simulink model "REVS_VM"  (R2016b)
settings: Solver=ode3  StartTime=REVS.sim_start_time_secs  StopTime=Inf  FixedStep=REVS.sim_step_time_secs  MaxStep=REVS.sim_step_time_secs  EnableMultiTasking=on
StopFcn:
  | postproc_datalog;
  | postproc_audit;
  | postproc_result;
model workspace (MATLAB code in the model file):
  other statements: REVS_setup_variants
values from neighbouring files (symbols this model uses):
  accessory = class_accessory_data    [class_test_data.m]
  battery = class_battery_data    [class_accessory_data.m]    (also in class_REVS_electric.m = class_REVS_battery)
  brake = struct(	'max_torque_Nm',[], 						'proportion_norm',1.0, 						'inertia_kgm2',0.0)    [class_REVS_drive_axle.m]
  engine = class_engine_data    [class_test_data.m]
  final_drive = struct(	'gear_ratio',[], 								'efficiency_norm',[], 								'inertia_kgm2',[] )    [class_REVS_drive_axle.m]
  gear = class_REVS_gearbox    [class_REVS_AT_transmission.m]
  tire = struct(	'radius_m',[], 						'rolling_resistance_coefficient',0, 						'vehicle_weight_norm',1.0,  						'wheel_slip_torque_Nm',[],  						'inertia_kgm2',0.0)    [class_REVS_drive_axle.m]
  torque_converter = class_REVS_torque_converter    [class_REVS_AT_transmission.m]
  transmission = class_transmission_data    [class_test_data.m]
  vehicle = class_vehicle_data    [class_test_data.m]
undefined symbols (not defined in the file or in its folder): alternator, ambient, controls, convert, DelayTimeSecs, drive_cycle, driver, electric, gear_strategy, InitialCondition, InitialValue, LoadSource, LookupStructure, MultiplyPosInputs, Normalize, NumPhases, REVS, SpeedSource, starter, tableshift, UpperSaturationLimit, Value, VerboseLevel, VerboseSignal
libraries: simulink x153
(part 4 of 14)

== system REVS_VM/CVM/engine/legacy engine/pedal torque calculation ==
  eng_on : Inport
  eng_spd_radps : Inport  Port=2
  eng_des_acl_norm : Inport  Port=3
  eng_des_load_limit_Nm : Inport  Port=4
  Closed Throttle Torque : Lookup_n-D  NumberOfTableDimensions=1  BreakpointsForDimension1=engine.closed_throttle_speed_radps  BeginIndexSearchUsingPreviousIndexResult=on  Table=engine.closed_throttle_torque_Nm  ExtrapMethod=Clip  UseLastTableValue=on  RndMeth=Simplest
  Full Throttle Torque : Lookup_n-D  NumberOfTableDimensions=1  BreakpointsForDimension1=engine.full_throttle_speed_radps  BeginIndexSearchUsingPreviousIndexResult=on  Table=engine.full_throttle_torque_Nm  ExtrapMethod=Clip  UseLastTableValue=on  RndMeth=Simplest
  MinMax5 : MinMax  Inputs=2  ZeroCross=off
  Pedal Map Torque : Lookup_n-D  BreakpointsForDimension1=engine.pedal_map_pedal_norm  BreakpointsForDimension2=engine.pedal_map_speed_radps  BeginIndexSearchUsingPreviousIndexResult=on  Table=engine.pedal_map_Nm  RndMeth=Simplest
  Product1 : Product
  Product2 : Product
  Product4 : Product  Inputs=3
  Sum : Sum
  to datalog1 : Subsystem
  to datalog2 : Subsystem
  to datalog3 : Subsystem
  to datalog4 : Subsystem
  to datalog5 : Subsystem
  des_pwr_W : Outport
  current_max_pwr_W : Outport  Port=2
  des_trq_Nm : Outport  Port=3
  current_max_trq_Nm : Outport  Port=4
  current_min_trq_Nm : Outport  Port=5
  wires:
  Pedal Map Torque/1 -> Product1/2
  eng_des_load_limit_Nm/1 -> MinMax5/2
  Full Throttle Torque/1 -> current_max_trq_Nm/1, to datalog4/1(Var), Product4/3
  Product4/1 -> current_max_pwr_W/1, to datalog3/1(Var)
  eng_spd_radps/1 -> Product2/1, Closed Throttle Torque/1, Full Throttle Torque/1, Product4/2, Pedal Map Torque/2
  Product2/1 -> to datalog2/1(Var), des_pwr_W/1
  MinMax5/1 -> to datalog1/1(Var), des_trq_Nm/1, Product2/2
  eng_on/1 -> Product4/1, Product1/1
  Closed Throttle Torque/1 -> Sum/1, current_min_trq_Nm/1, to datalog5/1(Var)
  Product1/1 -> Sum/2
  Sum/1 -> MinMax5/1
  eng_des_acl_norm/1 -> Pedal Map Torque/1

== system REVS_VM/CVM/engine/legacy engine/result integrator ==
  in : Inport
  Data Type Conversion : DataTypeConversion  OutDataTypeStr=double
  Integrator1 : Integrator  UpperSaturationLimit=Inf  LowerSaturationLimit=0  ZeroCross=off
  Integrator2 : Integrator  UpperSaturationLimit=Inf  LowerSaturationLimit=0  ZeroCross=off
  Phase To Workspace : ToWorkspace  VariableName=result__phase_fuel_consumed_g  SampleTime=-1
  Product1 : Product  Multiplication=Matrix(*)
  Reshape : Reshape
  Total To Workspace : ToWorkspace  VariableName=result__total_fuel_consumed_g  SampleTime=-1
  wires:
  Reshape/1 -> Integrator1/1, Product1/1
  Data Type Conversion/1 -> Reshape/1
  Integrator2/1 -> Phase To Workspace/1
  [REVS_phase_flag] -> Product1/2
  Product1/1 -> Integrator2/1
  Integrator1/1 -> Total To Workspace/1
  in/1 -> Data Type Conversion/1

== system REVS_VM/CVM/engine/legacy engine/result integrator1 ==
  in : Inport
  Data Type Conversion : DataTypeConversion  OutDataTypeStr=double
  Integrator1 : Integrator  UpperSaturationLimit=Inf  LowerSaturationLimit=0  ZeroCross=off
  Integrator2 : Integrator  UpperSaturationLimit=Inf  LowerSaturationLimit=0  ZeroCross=off
  Phase To Workspace : ToWorkspace  VariableName=result__phase_engine_revolutions  SampleTime=-1
  Product1 : Product  Multiplication=Matrix(*)
  Reshape : Reshape
  Total To Workspace : ToWorkspace  VariableName=result__total_engine_revolutions  SampleTime=-1
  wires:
  Reshape/1 -> Integrator1/1, Product1/1
  Data Type Conversion/1 -> Reshape/1
  Integrator2/1 -> Phase To Workspace/1
  [REVS_phase_flag] -> Product1/2
  Product1/1 -> Integrator2/1
  Integrator1/1 -> Total To Workspace/1
  in/1 -> Data Type Conversion/1

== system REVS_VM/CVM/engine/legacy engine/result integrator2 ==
  in : Inport
  Data Type Conversion : DataTypeConversion  OutDataTypeStr=double
  Integrator1 : Integrator  UpperSaturationLimit=Inf  LowerSaturationLimit=0  ZeroCross=off
  Integrator2 : Integrator  UpperSaturationLimit=Inf  LowerSaturationLimit=0  ZeroCross=off
  Phase To Workspace : ToWorkspace  VariableName=result__phase_engine_running_time_secs  SampleTime=-1
  Product1 : Product  Multiplication=Matrix(*)
  Reshape : Reshape
  Total To Workspace : ToWorkspace  VariableName=result__total_engine_running_time_secs  SampleTime=-1
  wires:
  Reshape/1 -> Integrator1/1, Product1/1
  Data Type Conversion/1 -> Reshape/1
  Integrator2/1 -> Phase To Workspace/1
  [REVS_phase_flag] -> Product1/2
  Product1/1 -> Integrator2/1
  Integrator1/1 -> Total To Workspace/1
  in/1 -> Data Type Conversion/1

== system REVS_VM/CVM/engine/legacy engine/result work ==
  torque_Nm : Inport
  speed_radps : Inport  Port=2
  upstream_iner_kgm2 : Inport  Port=3
  Derivative : Derivative  CoefficientInTFapproximation=1e6
  Gain : Gain  Gain=1/1000
  Integrator1 : Integrator  UpperSaturationLimit=Inf  LowerSaturationLimit=0  ZeroCross=off
  Integrator2 : Integrator  UpperSaturationLimit=Inf  LowerSaturationLimit=0  ZeroCross=off
  Phase To Workspace : ToWorkspace  VariableName=result__phase_crankshaft_output_pos_work_kJ  SampleTime=-1
  Pos : Fcn  Expr=u(1)*(u(1) >= 0)
  Product : Product
  Product1 : Product
  Product2 : Product
  Subtract : Sum  Inputs=+-
  Total To Workspace : ToWorkspace  VariableName=result__total_crankshaft_output_pos_work_kJ  SampleTime=-1
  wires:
  Product2/1 -> Pos/1
  Pos/1 -> Gain/1
  Gain/1 -> Integrator1/1, Product/2
  Product1/1 -> Subtract/2
  Derivative/1 -> Product1/1
  speed_radps/1 -> Derivative/1, Product2/2
  upstream_iner_kgm2/1 -> Product1/2
  Subtract/1 -> Product2/1
  Integrator2/1 -> Phase To Workspace/1
  [REVS_phase_flag] -> Product/1
  Product/1 -> Integrator2/1
  Integrator1/1 -> Total To Workspace/1
  torque_Nm/1 -> Subtract/1

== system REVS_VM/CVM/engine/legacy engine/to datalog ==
  Var : Inport
  Constant : Constant  Value=VerboseSignal
  Constant1 : Constant  Value=VerboseLevel
  Relational Operator : RelationalOperator  OutDataTypeStr=boolean  ZeroCross=off
  Subsystem : Subsystem
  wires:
  Constant1/1 -> Relational Operator/2
  Constant/1 -> Relational Operator/1
  Relational Operator/1 -> Subsystem/Enable
  Var/1 -> Subsystem/1(In1)

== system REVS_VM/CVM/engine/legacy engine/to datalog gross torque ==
  Var : Inport
  Constant : Constant  Value=VerboseSignal
  Constant1 : Constant  Value=VerboseLevel
  Relational Operator : RelationalOperator  OutDataTypeStr=boolean  ZeroCross=off
  Subsystem : Subsystem
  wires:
  Constant1/1 -> Relational Operator/2
  Constant/1 -> Relational Operator/1
  Relational Operator/1 -> Subsystem/Enable
  Var/1 -> Subsystem/1(In1)

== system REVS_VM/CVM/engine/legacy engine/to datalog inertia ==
  Var : Inport
  Constant : Constant  Value=VerboseSignal
  Constant1 : Constant  Value=VerboseLevel
  Relational Operator : RelationalOperator  OutDataTypeStr=boolean  ZeroCross=off
  Subsystem : Subsystem
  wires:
  Constant1/1 -> Relational Operator/2
  Constant/1 -> Relational Operator/1
  Relational Operator/1 -> Subsystem/Enable
  Var/1 -> Subsystem/1(In1)

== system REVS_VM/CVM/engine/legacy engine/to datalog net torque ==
  Var : Inport
  Constant : Constant  Value=VerboseSignal
  Constant1 : Constant  Value=VerboseLevel
  Relational Operator : RelationalOperator  OutDataTypeStr=boolean  ZeroCross=off
  Subsystem : Subsystem
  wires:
  Constant1/1 -> Relational Operator/2
  Constant/1 -> Relational Operator/1
  Relational Operator/1 -> Subsystem/Enable
  Var/1 -> Subsystem/1(In1)

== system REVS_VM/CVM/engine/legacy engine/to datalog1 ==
  Var : Inport
  Constant : Constant  Value=VerboseSignal
  Constant1 : Constant  Value=VerboseLevel
  Relational Operator : RelationalOperator  OutDataTypeStr=boolean  ZeroCross=off
  Subsystem : Subsystem
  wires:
  Constant1/1 -> Relational Operator/2
  Constant/1 -> Relational Operator/1
  Relational Operator/1 -> Subsystem/Enable
  Var/1 -> Subsystem/1(In1)

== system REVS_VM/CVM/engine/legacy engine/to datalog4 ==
  Var : Inport
  Constant : Constant  Value=VerboseSignal
  Constant1 : Constant  Value=VerboseLevel
  Relational Operator : RelationalOperator  OutDataTypeStr=boolean  ZeroCross=off
  Subsystem : Subsystem
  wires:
  Constant1/1 -> Relational Operator/2
  Constant/1 -> Relational Operator/1
  Relational Operator/1 -> Subsystem/Enable
  Var/1 -> Subsystem/1(In1)

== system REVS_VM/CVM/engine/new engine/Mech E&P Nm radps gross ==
  " trq_Nm" : Inport
  spd_radps : Inport  Port=2
  iner_kgm2 : Inport  Port=3
  Compare To Constant : simulink/Logic and Bit Operations/Compare To Constant  relop=>=  const=1  OutDataTypeStr=boolean
  Constant : Constant  Value=VerboseSignal
  Subsystem : Subsystem
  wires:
  Constant/1 -> Compare To Constant/1
  Compare To Constant/1 -> Subsystem/Enable
  iner_kgm2/1 -> Subsystem/3(iner_kgm2)
  spd_radps/1 -> Subsystem/2(spd_radps)
  " trq_Nm"/1 -> Subsystem/1(" trq_Nm")

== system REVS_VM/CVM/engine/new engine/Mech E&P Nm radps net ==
  " trq_Nm" : Inport
  spd_radps : Inport  Port=2
  iner_kgm2 : Inport  Port=3
  Compare To Constant : simulink/Logic and Bit Operations/Compare To Constant  relop=>=  const=1  OutDataTypeStr=boolean
  Constant : Constant  Value=VerboseSignal
  Subsystem : Subsystem
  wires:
  Constant/1 -> Compare To Constant/1
  Compare To Constant/1 -> Subsystem/Enable
  iner_kgm2/1 -> Subsystem/3(iner_kgm2)
  spd_radps/1 -> Subsystem/2(spd_radps)
  " trq_Nm"/1 -> Subsystem/1(" trq_Nm")

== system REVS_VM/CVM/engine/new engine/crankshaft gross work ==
  torque_Nm : Inport
  speed_radps : Inport  Port=2
  upstream_iner_kgm2 : Inport  Port=3
  Derivative : Derivative  CoefficientInTFapproximation=1e6
  Gain : Gain  Gain=1/1000
  Integrator1 : Integrator  UpperSaturationLimit=Inf  LowerSaturationLimit=0  ZeroCross=off
  Integrator2 : Integrator  UpperSaturationLimit=Inf  LowerSaturationLimit=0  ZeroCross=off
  Phase To Workspace : ToWorkspace  VariableName=result__phase_crankshaft_gross_pos_work_kJ  SampleTime=-1
  Pos : Fcn  Expr=u(1)*(u(1) >= 0)
  Product : Product
  Product1 : Product
  Product2 : Product
  Subtract : Sum  Inputs=+-
  Total To Workspace : ToWorkspace  VariableName=result__total_crankshaft_gross_pos_work_kJ  SampleTime=-1
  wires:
  Product2/1 -> Pos/1
  Pos/1 -> Gain/1
  Gain/1 -> Integrator1/1, Product/2
  Product1/1 -> Subtract/2
  Derivative/1 -> Product1/1
  speed_radps/1 -> Derivative/1, Product2/2
  upstream_iner_kgm2/1 -> Product1/2
  Subtract/1 -> Product2/1
  Integrator2/1 -> Phase To Workspace/1
  [REVS_phase_flag] -> Product/1
  Product/1 -> Integrator2/1
  Integrator1/1 -> Total To Workspace/1
  torque_Nm/1 -> Subtract/1

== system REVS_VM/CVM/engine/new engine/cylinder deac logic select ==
  note: 1) Only subsystems can be added as variant choices at this level 2) Blocks cannot be connected at this level as connectivity is automatically determined at simulation, based on the active variant
  system_bus : Inport
  constant : Subsystem  VariantControl=get_REVS_engine_deac_strategy_type( engine) == enum_engine_deac_select.constant
  dynamic criteria : Subsystem  VariantControl=get_REVS_engine_deac_strategy_type( engine) == enum_engine_deac_select.dynamic_criteria
  dynamic lookup : Subsystem  VariantControl="get_REVS_engine_deac_strategy_type( engine) ==  enum_engine_deac_select.dynamic_lookup"
  cyl_deac_norm : Outport

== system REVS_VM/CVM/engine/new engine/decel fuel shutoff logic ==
  system_bus : Inport
  eng_rqst_torque_Nm : Inport  Port=2
  eng_load_norm : Inport  Port=3
  Constant : Constant  Value=engine.max_torque_Nm
  Divide : Product  Inputs=*/
  Logical Operator : Logic  Inputs=3  AllPortsSameDT=off  OutDataTypeStr=boolean
  Relay : Relay  OnSwitchValue=0.01  OffSwitchValue=0.005  OnOutputValue=0  OffOutputValue=1  ZeroCross=off
  Relay1 : Relay  OnSwitchValue=0.01  OffSwitchValue=0.005  OnOutputValue=0  OffOutputValue=1  ZeroCross=off
  dynamic equation : Subsystem
  to datalog4 : Subsystem
  dfco_active_bool : Outport
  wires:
  Relay1/1 -> Logical Operator/3
  eng_load_norm/1 -> Relay1/1
  Divide/1 -> Relay/1
  Constant/1 -> Divide/2
  eng_rqst_torque_Nm/1 -> Divide/1
  Relay/1 -> Logical Operator/2
  Logical Operator/1 -> dfco_active_bool/1, to datalog4/1(Var)
  system_bus/1 -> dynamic equation/1(bus)
  dynamic equation/1(out) -> Logical Operator/1

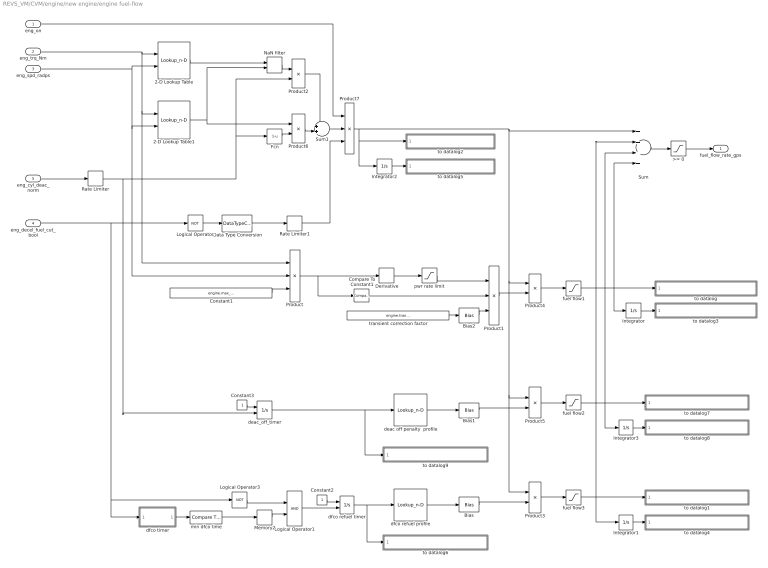
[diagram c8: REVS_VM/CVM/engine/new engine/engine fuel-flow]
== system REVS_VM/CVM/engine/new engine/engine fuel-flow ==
  eng_on : Inport
  eng_trq_Nm : Inport  Port=2
  eng_spd_radps : Inport  Port=3
  eng_decel_fuel_cut_bool : Inport  Port=4
  eng_cyl_deac_norm : Inport  Port=5
  2-D Lookup Table : Lookup_n-D  BreakpointsForDimension1=engine.fuel_map_torque_Nm  BreakpointsForDimension2=engine.fuel_map_speed_radps  IndexSearchMethod=Linear search  BeginIndexSearchUsingPreviousIndexResult=on  Table=engine.deac_fuel_map_gps  ExtrapMethod=Clip  UseLastTableValue=on  RndMeth=Simplest
  2-D Lookup Table1 : Lookup_n-D  BreakpointsForDimension1=engine.fuel_map_torque_Nm  BreakpointsForDimension2=engine.fuel_map_speed_radps  IndexSearchMethod=Linear search  BeginIndexSearchUsingPreviousIndexResult=on  Table=engine.fuel_map_gps  ExtrapMethod=Clip  UseLastTableValue=on  RndMeth=Simplest
  >= 0 : Saturate  UpperLimit=Inf  LowerLimit=0  ZeroCross=off
  Bias : Bias  Bias=-1
  Bias1 : Bias  Bias=-1
  Bias2 : Bias  Bias=-1
  Compare To Constant1 : simulink/Logic and Bit Operations/Compare To Constant  relop=>  const=0  OutDataTypeStr=boolean  ZeroCross=off
  Constant1 : Constant  Value=engine.max_power_W
  Constant2 : Constant
  Constant3 : Constant
  Data Type Conversion : DataTypeConversion  OutDataTypeStr=double
  Derivative : Derivative
  Fcn : Fcn  Expr=1-u
  Integrator{,1..3} (4 alike) : Integrator
  Logical Operator : Logic  Operator=NOT  AllPortsSameDT=off  OutDataTypeStr=boolean
  Logical Operator3 : Logic  Operator=NOT  AllPortsSameDT=off  OutDataTypeStr=boolean
  Logical Operator1 : Logic  AllPortsSameDT=off  OutDataTypeStr=boolean
  Memory2 : Memory
  NaN filter : MinMax  Inputs=2
  Product : Product  Inputs=**/
  Product1 : Product  Inputs=3
  Product{2..6} (5 alike) : Product
  Product7 : Product  Inputs=3
  Rate Limiter : RateLimiter  RisingSlewLimit=1/engine.deac_transition_on_duration_secs  FallingSlewLimit=-1/engine.deac_transition_off_duration_secs  SampleTimeMode=inherited
  Rate Limiter1 : RateLimiter  RisingSlewLimit=5  FallingSlewLimit=-3  SampleTimeMode=inherited
  Sum : Sum  Inputs=++++
  Sum1 : Sum  Inputs=++|
  deac off penalty  profile : Lookup_n-D  NumberOfTableDimensions=1  BreakpointsForDimension1=engine.deac_transition_off_fuel_multiplier_time_secs  IndexSearchMethod=Linear search  BeginIndexSearchUsingPreviousIndexResult=on  Table=engine.deac_transition_off_fuel_multiplier  ExtrapMethod=Clip  RndMeth=Simplest
  deac_off_timer : Integrator  ExternalReset=level
  dfco refuel timer : Integrator  ExternalReset=rising
  dfco refuel profile : Lookup_n-D  NumberOfTableDimensions=1  BreakpointsForDimension1=engine.DFCO_refuel_multiplier_time_secs  IndexSearchMethod=Linear search  BeginIndexSearchUsingPreviousIndexResult=on  Table=engine.DFCO_refuel_multiplier  ExtrapMethod=Clip  RndMeth=Simplest
  dfco timer : Subsystem
  fuel flow1 : Saturate  UpperLimit=inf  LowerLimit=0  ZeroCross=off
  fuel flow2 : Saturate  UpperLimit=engine.deac_transition_off_fuel_multiplier_limit_gps  LowerLimit=0  ZeroCross=off
  fuel flow3 : Saturate  UpperLimit=engine.DFCO_refuel_multiplier_limit_gps  LowerLimit=0  ZeroCross=off
  min dfco time : simulink/Logic and Bit Operations/Compare To Constant  relop=>=  const=engine.DFCO_min_duration_secs  OutDataTypeStr=boolean  ZeroCross=off
  pwr rate limit : Saturate  UpperLimit=0.4  LowerLimit=0  ZeroCross=off
  to datalog : Subsystem
  to datalog1 : Subsystem
  to datalog2 : Subsystem
  to datalog3 : Subsystem
  to datalog4 : Subsystem
  to datalog5 : Subsystem
  to datalog6 : Subsystem
  to datalog7 : Subsystem
  to datalog8 : Subsystem
  to datalog9 : Subsystem
  transient correction factor : Constant  Value=engine.transient_correction_mult
  fuel_flow_rate_gps : Outport
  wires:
  Data Type Conversion/1 -> Rate Limiter1/1
  Rate Limiter1/1 -> Product7/3
  eng_cyl_deac_norm/1 -> Rate Limiter/1
  Bias1/1 -> Product5/2
  deac_off_timer/1 -> deac off penalty  profile/1, to datalog9/1(Var)
  Rate Limiter/1 -> deac_off_timer/2, Fcn/1, Product2/2
  Constant3/1 -> deac_off_timer/1
  deac off penalty  profile/1 -> Bias1/1
  Integrator3/1 -> to datalog8/1(Var)
  Product7/1 -> Integrator2/1, to datalog2/1(Var), Sum/1, Product4/1, Product3/1, Product5/1
  Product5/1 -> fuel flow2/1
  fuel flow2/1 -> to datalog7/1(Var), Sum/3, Integrator3/1
  Sum1/1 -> Product7/2
  Logical Operator3/1 -> Logical Operator1/1
  Logical Operator/1 -> Data Type Conversion/1
  NaN filter/1 -> Product2/1
  Fcn/1 -> Product6/2
  Product2/1 -> Sum1/1
  Product6/1 -> Sum1/2
  2-D Lookup Table1/1 -> NaN filter/2, Product6/1
  Bias/1 -> Product3/2
  dfco refuel profile/1 -> Bias/1
  dfco refuel timer/1 -> dfco refuel profile/1, to datalog6/1(Var)
  Constant2/1 -> dfco refuel timer/1
  Integrator2/1 -> to datalog5/1(Var)
  Derivative/1 -> pwr rate limit/1
  Constant1/1 -> Product/3
  Bias2/1 -> Product1/3
  Product1/1 -> Product4/2
  Integrator1/1 -> to datalog4/1(Var)
  Integrator/1 -> to datalog3/1(Var)
  fuel flow1/1 -> Integrator/1, to datalog/1(Var), Sum/4
  Product4/1 -> fuel flow1/1
  transient correction factor/1 -> Bias2/1
  pwr rate limit/1 -> Product1/1
  Product/1 -> Derivative/1, Compare To Constant1/1
  eng_trq_Nm/1 -> 2-D Lookup Table/1, 2-D Lookup Table1/1, Product/1
  Compare To Constant1/1 -> Product1/2
  eng_spd_radps/1 -> 2-D Lookup Table/2, 2-D Lookup Table1/2, Product/2
  eng_on/1 -> Product7/1
  2-D Lookup Table/1 -> NaN filter/1
  >= 0/1 -> fuel_flow_rate_gps/1
  dfco timer/1(out) -> min dfco time/1
  min dfco time/1 -> Memory2/1
  Memory2/1 -> Logical Operator1/2
  Logical Operator1/1 -> dfco refuel timer/2
  Sum/1 -> >= 0/1
  Product3/1 -> fuel flow3/1
  fuel flow3/1 -> to datalog1/1(Var), Sum/2, Integrator1/1
  eng_decel_fuel_cut_bool/1 -> Logical Operator/1, Logical Operator3/1, dfco timer/1(bool)

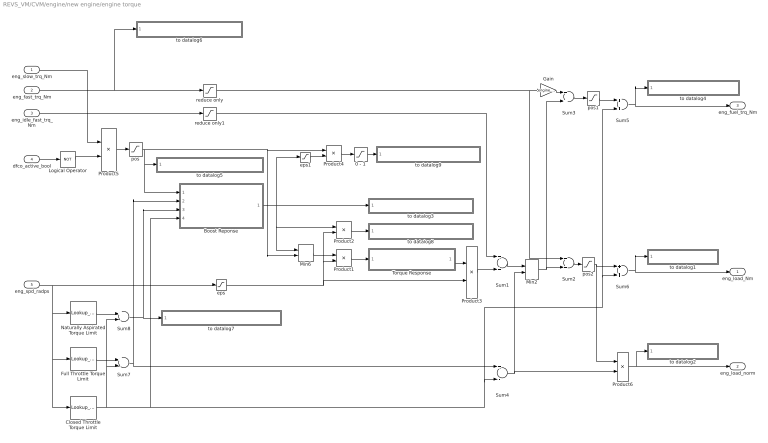
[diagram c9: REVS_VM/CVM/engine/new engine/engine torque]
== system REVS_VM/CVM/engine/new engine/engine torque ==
  eng_slow_trq_Nm : Inport
  eng_fast_trq_Nm : Inport  Port=2
  eng_idle_fast_trq_Nm : Inport  Port=3
  dfco_active_bool : Inport  Port=4
  eng_spd_radps : Inport  Port=5
  0 - 1 : Saturate  UpperLimit=1  LowerLimit=0  ZeroCross=off
  Boost Reponse : Subsystem
  Closed Throttle Torque Limit : Lookup_n-D  NumberOfTableDimensions=1  BreakpointsForDimension1=engine.closed_throttle_speed_radps  BeginIndexSearchUsingPreviousIndexResult=on  Table=engine.closed_throttle_torque_Nm  ExtrapMethod=Clip  UseLastTableValue=on  RndMeth=Simplest
  Full Throttle Torque Limit : Lookup_n-D  NumberOfTableDimensions=1  BreakpointsForDimension1=engine.full_throttle_speed_radps  BeginIndexSearchUsingPreviousIndexResult=on  Table=engine.full_throttle_torque_Nm  ExtrapMethod=Clip  UseLastTableValue=on  RndMeth=Simplest
  Gain : Gain  Gain=engine.fast_torque_fuel_adjust_norm
  Logical Operator : Logic  Operator=NOT  AllPortsSameDT=off  OutDataTypeStr=boolean
  Min2 : MinMax  Inputs=2  ZeroCross=off
  Min6 : MinMax  Inputs=2  ZeroCross=off
  Naturally Aspirated Torque Limit : Lookup_n-D  NumberOfTableDimensions=1  BreakpointsForDimension1=engine.naturally_aspirated_speed_radps  IndexSearchMethod=Linear search  BeginIndexSearchUsingPreviousIndexResult=on  Table=engine.naturally_aspirated_torque_Nm  ExtrapMethod=Clip  UseLastTableValue=on  RndMeth=Simplest
  Product1 : Product
  Product2 : Product
  Product3 : Product  Inputs=*/
  Product4 : Product  Inputs=*/
  Product5 : Product
  Product6 : Product  Inputs=*/
  Sum{1..3,5..6} (5 alike) : Sum
  Sum4 : Sum  Inputs=+-
  Sum7 : Sum  Inputs=+-
  Sum8 : Sum  Inputs=+-
  Torque Response : Subsystem
  eps : Saturate  UpperLimit=inf  LowerLimit=eps
  eps1 : Saturate  UpperLimit=inf  LowerLimit=eps
  pos : Saturate  UpperLimit=inf  LowerLimit=0  ZeroCross=off
  pos1 : Saturate  UpperLimit=inf  LowerLimit=0  ZeroCross=off
  pos2 : Saturate  UpperLimit=inf  LowerLimit=0  ZeroCross=off
  reduce only : Saturate  UpperLimit=0  LowerLimit=-inf  ZeroCross=off
  reduce only1 : Saturate  UpperLimit=0  LowerLimit=-inf  ZeroCross=off
  to datalog1 : Subsystem
  to datalog2 : Subsystem
  to datalog3 : Subsystem
  to datalog4 : Subsystem
  to datalog5 : Subsystem
  to datalog6 : Subsystem
  to datalog7 : Subsystem
  to datalog8 : Subsystem
  to datalog9 : Subsystem
  eng_load_Nm : Outport
  eng_load_norm : Outport  Port=2
  eng_fuel_trq_Nm : Outport  Port=3
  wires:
  pos2/1 -> Product6/1, Sum6/1
  pos1/1 -> Sum5/1
  Sum4/1 -> Product6/2, Min2/2
  Torque Response/1(act_pow_W) -> Product3/1
  Sum3/1 -> pos1/1
  Sum2/1 -> pos2/1
  Logical Operator/1 -> Product5/2
  Product5/1 -> pos/1
  Min2/1 -> Sum2/2, Sum3/2
  dfco_active_bool/1 -> Logical Operator/1
  0 - 1/1 -> to datalog9/1(Var)
  eps1/1 -> Product4/2
  Min6/1 -> Product1/1
  eng_slow_trq_Nm/1 -> Product5/1
  reduce only1/1 -> Sum1/1
  eng_idle_fast_trq_Nm/1 -> reduce only1/1
  Product4/1 -> 0 - 1/1
  eps/1 -> Product1/2, Product2/2, Product3/2
  Product1/1 -> Torque Response/1(target_pow_W)
  Product2/1 -> to datalog8/1(Var)
  Product6/1 -> to datalog2/1(Var), eng_load_norm/1
  Closed Throttle Torque Limit/1 -> Sum8/2, Sum7/2, Sum6/2, Sum5/2, Sum4/2, Boost Reponse/4(min_trq_Nm)
  Sum7/1 -> Sum4/1, Boost Reponse/2(max_trq_Nm)
  Sum8/1 -> Boost Reponse/3(nat_asp_trq_Nm), to datalog7/1(Var)
  pos/1 -> Min6/2, Product4/1, to datalog5/1(Var), Boost Reponse/1(target_trq_Nm)
  Product3/1 -> Sum1/2
  Gain/1 -> Sum3/1
  Sum5/1 -> to datalog4/1(Var), eng_fuel_trq_Nm/1
  Sum1/1 -> Min2/1
  reduce only/1 -> Sum2/1, Gain/1
  eng_fast_trq_Nm/1 -> reduce only/1, to datalog6/1(Var)
  eng_spd_radps/1 -> eps/1, Closed Throttle Torque Limit/1, Full Throttle Torque Limit/1, Naturally Aspirated Torque Limit/1
  Sum6/1 -> to datalog1/1(Var), eng_load_Nm/1
  Boost Reponse/1(trq_limit_Nm) -> to datalog3/1(Var), eps1/1, Product2/1, Min6/1
  Full Throttle Torque Limit/1 -> Sum7/1
  Naturally Aspirated Torque Limit/1 -> Sum8/1

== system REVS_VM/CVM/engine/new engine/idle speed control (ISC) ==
  system_bus : Inport
  eng_spd_radps : Inport  Port=2
  Add : Sum  Inputs=++-
  Closed Throttle Torque : Lookup_n-D  NumberOfTableDimensions=1  BreakpointsForDimension1=engine.closed_throttle_speed_radps  IndexSearchMethod=Linear search  BeginIndexSearchUsingPreviousIndexResult=on  Table=engine.closed_throttle_torque_Nm  ExtrapMethod=Clip  UseLastTableValue=on  RndMeth=Simplest
  Derivative : Derivative
  ISC state : Subsystem
  Idle Speed Target : Subsystem
  PID control : Subsystem
  Split Control Torque : Subsystem
  Sum1 : Sum  Inputs=+-|
  Sum2 : Sum  Inputs=+-
  Taper : Lookup_n-D  NumberOfTableDimensions=1  BreakpointsForDimension1=[-20,-10,0,5,10,15,20]  IndexSearchMethod=Linear search  BeginIndexSearchUsingPreviousIndexResult=on  Table=[-20,-10,0,5,8,10,10]  UseLastTableValue=on  RndMeth=Simplest
  driver bus1 : BusSelector  OutputSignals=powertrain.control.ctrl_eng_on,powertrain.trans.ctrl.eng_des_spd_radps
  eng iner : Gain  Gain=engine.inertia_kgm2
  eng iner2 : Gain  Gain=engine.inertia_kgm2
  gain : Gain  Gain=0.8
  to datalog4 : Subsystem
  to datalog5 : Subsystem
  to datalog6 : Subsystem
  to datalog7 : Subsystem
  to datalog8 : Subsystem
  ISC_state : Outport
  ISC_target_spd_radps : Outport  Port=2
  ISC_slow_trq_Nm : Outport  Port=3
  "ISC_fast_trq_Nm " : Outport  Port=4
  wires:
  Sum1/1 -> Taper/1
  Closed Throttle Torque/1 -> gain/1
  Derivative/1 -> eng iner2/1
  PID control/1(PID_trq_Nm) -> Add/1
  eng iner/1 -> PID control/2(error)
  Add/1 -> Split Control Torque/2(ISC_trq)
  Split Control Torque/2(ISC_fast_trq) -> to datalog8/1(Var), "ISC_fast_trq_Nm "/1
  Split Control Torque/1(ISC_slow_trq) -> ISC_slow_trq_Nm/1, to datalog7/1(Var)
  driver bus1/1 -> ISC state/1(eng_on)  "<ctrl_eng_on>"
  system_bus/1 -> Idle Speed Target/1(system_bus), driver bus1/1
  driver bus1/2 -> Idle Speed Target/3(eng_des_spd_radps)  "<eng_des_spd_radps>"
  ISC state/1(state) -> Idle Speed Target/4(ISC_state), PID control/1(ISC_state), Split Control Torque/1(ISC_state), to datalog6/1(Var), ISC_state/1
  Sum2/1 -> eng iner/1
  eng_spd_radps/1 -> Sum1/2, Closed Throttle Torque/1, Sum2/2, Idle Speed Target/2(eng_spd_radps), ISC state/2(eng_spd_radps)
  Idle Speed Target/1(target_idle_spd_radps) -> Sum1/1, to datalog5/1(Var), ISC_target_spd_radps/1, Sum2/1
  Taper/1 -> Derivative/1
  gain/1 -> Add/3
  eng iner2/1 -> to datalog4/1(Var), Add/2

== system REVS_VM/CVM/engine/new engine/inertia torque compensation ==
  eng_on : Inport
  comp_iner_enable : Inport  Port=2
  eng_spd_radps : Inport  Port=3
  iner_kgm2 : Inport  Port=4
  load_norm : Inport  Port=5
  <= 0 : Saturate  UpperLimit=0  LowerLimit=-Inf  ZeroCross=off
  Memory : Memory
  Product : Product  Inputs=5
  Transfer Fcn : TransferFcn  Numerator=[1 0]  Denominator=[0.02 1]
  downstream compensation : Gain  Gain=1.5
  load based inertia adj. norm : Lookup_n-D  NumberOfTableDimensions=1  BreakpointsForDimension1=[0, 0.65, 0.90, 1.0]  Table=[1.0, 1.0, 0.0, 0.0]  InternalRulePriority=Speed  RndMeth=Simplest
  to datalog1 : Subsystem
  comp_trq_Nm : Outport
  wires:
  comp_iner_enable/1 -> Product/2
  downstream compensation/1 -> Product/4
  Transfer Fcn/1 -> Product/3
  eng_spd_radps/1 -> Transfer Fcn/1
  iner_kgm2/1 -> downstream compensation/1
  <= 0/1 -> to datalog1/1(Var), comp_trq_Nm/1
  eng_on/1 -> Product/1
  load_norm/1 -> Memory/1
  Memory/1 -> load based inertia adj. norm/1
  load based inertia adj. norm/1 -> Product/5
  Product/1 -> <= 0/1

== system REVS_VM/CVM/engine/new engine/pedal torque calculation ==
  eng_on : Inport
  eng_des_acl_norm : Inport  Port=2
  eng_des_load_limit_Nm : Inport  Port=3
  eng_spd_radps : Inport  Port=4
  Closed Throttle Torque : Lookup_n-D  NumberOfTableDimensions=1  BreakpointsForDimension1=engine.closed_throttle_speed_radps  BeginIndexSearchUsingPreviousIndexResult=on  Table=engine.closed_throttle_torque_Nm  ExtrapMethod=Clip  UseLastTableValue=on  RndMeth=Simplest
  MinMax5 : MinMax  Inputs=2  ZeroCross=off
  Pedal Map Torque : Lookup_n-D  BreakpointsForDimension1=engine.pedal_map_pedal_norm  BreakpointsForDimension2=engine.pedal_map_speed_radps  BeginIndexSearchUsingPreviousIndexResult=on  Table=engine.pedal_map_Nm  RndMeth=Simplest
  Product1 : Product
  Product2 : Product
  Sum : Sum
  to datalog1 : Subsystem
  to datalog2 : Subsystem
  to datalog3 : Subsystem
  des_pwr_W : Outport
  des_trq_Nm : Outport  Port=2
  des_gross_trq_Nm : Outport  Port=3
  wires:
  eng_des_load_limit_Nm/1 -> MinMax5/2
  Product1/1 -> MinMax5/1
  MinMax5/1 -> Sum/2, des_gross_trq_Nm/1, to datalog3/1(Var)
  eng_des_acl_norm/1 -> Pedal Map Torque/1
  Closed Throttle Torque/1 -> Sum/1
  eng_on/1 -> Product1/1
  Sum/1 -> des_trq_Nm/1, to datalog1/1(Var), Product2/2
  Product2/1 -> des_pwr_W/1, to datalog2/1(Var)
  eng_spd_radps/1 -> Pedal Map Torque/2, Closed Throttle Torque/1, Product2/1
  Pedal Map Torque/1 -> Product1/2

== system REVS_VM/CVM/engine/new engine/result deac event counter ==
  in : Inport
  Data Type Conversion : DataTypeConversion  OutDataTypeStr=double
  Phase Memory : Memory
  Phase To Workspace : ToWorkspace  VariableName=result__phase_engine_deac_events  SampleTime=-1
  Product : Product
  Sum : Sum  Inputs=|++
  Sum1 : Sum  Inputs=|++
  Total Memory : Memory
  Total To Workspace : ToWorkspace  VariableName=result__total_engine_deac_events  SampleTime=-1
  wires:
  Data Type Conversion/1 -> Product/2, Sum1/1
  Sum1/1 -> Total Memory/1
  Sum/1 -> Phase Memory/1
  in/1 -> Data Type Conversion/1
  Total Memory/1 -> Sum1/2, Total To Workspace/1
  Product/1 -> Sum/1
  [REVS_phase_flag] -> Product/1
  Phase Memory/1 -> Phase To Workspace/1, Sum/2

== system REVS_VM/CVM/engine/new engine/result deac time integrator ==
  in : Inport
  Data Type Conversion : DataTypeConversion  OutDataTypeStr=double
  Integrator1 : Integrator  UpperSaturationLimit=Inf  LowerSaturationLimit=0  ZeroCross=off
  Integrator2 : Integrator  UpperSaturationLimit=Inf  LowerSaturationLimit=0  ZeroCross=off
  Phase To Workspace : ToWorkspace  VariableName=result__phase_engine_deac_time_secs  SampleTime=-1
  Product1 : Product  Multiplication=Matrix(*)
  Reshape : Reshape
  Total To Workspace : ToWorkspace  VariableName=result__total_engine_deac_time_secs  SampleTime=-1
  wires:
  Reshape/1 -> Integrator1/1, Product1/1
  Data Type Conversion/1 -> Reshape/1
  Integrator2/1 -> Phase To Workspace/1
  [REVS_phase_flag] -> Product1/2
  Product1/1 -> Integrator2/1
  Integrator1/1 -> Total To Workspace/1
  in/1 -> Data Type Conversion/1

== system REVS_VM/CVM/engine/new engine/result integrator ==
  in : Inport
  Data Type Conversion : DataTypeConversion  OutDataTypeStr=double
  Integrator1 : Integrator  UpperSaturationLimit=Inf  LowerSaturationLimit=0  ZeroCross=off
  Integrator2 : Integrator  UpperSaturationLimit=Inf  LowerSaturationLimit=0  ZeroCross=off
  Phase To Workspace : ToWorkspace  VariableName=result__phase_fuel_consumed_g  SampleTime=-1
  Product1 : Product  Multiplication=Matrix(*)
  Reshape : Reshape
  Total To Workspace : ToWorkspace  VariableName=result__total_fuel_consumed_g  SampleTime=-1
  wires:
  Reshape/1 -> Integrator1/1, Product1/1
  Data Type Conversion/1 -> Reshape/1
  Integrator2/1 -> Phase To Workspace/1
  [REVS_phase_flag] -> Product1/2
  Product1/1 -> Integrator2/1
  Integrator1/1 -> Total To Workspace/1
  in/1 -> Data Type Conversion/1

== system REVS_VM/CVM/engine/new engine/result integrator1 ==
  in : Inport
  Data Type Conversion : DataTypeConversion  OutDataTypeStr=double
  Integrator1 : Integrator  UpperSaturationLimit=Inf  LowerSaturationLimit=0  ZeroCross=off
  Integrator2 : Integrator  UpperSaturationLimit=Inf  LowerSaturationLimit=0  ZeroCross=off
  Phase To Workspace : ToWorkspace  VariableName=result__phase_engine_revolutions  SampleTime=-1
  Product1 : Product  Multiplication=Matrix(*)
  Reshape : Reshape
  Total To Workspace : ToWorkspace  VariableName=result__total_engine_revolutions  SampleTime=-1
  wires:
  Reshape/1 -> Integrator1/1, Product1/1
  Data Type Conversion/1 -> Reshape/1
  Integrator2/1 -> Phase To Workspace/1
  [REVS_phase_flag] -> Product1/2
  Product1/1 -> Integrator2/1
  Integrator1/1 -> Total To Workspace/1
  in/1 -> Data Type Conversion/1

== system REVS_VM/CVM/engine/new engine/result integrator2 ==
  in : Inport
  Data Type Conversion : DataTypeConversion  OutDataTypeStr=double
  Integrator1 : Integrator  UpperSaturationLimit=Inf  LowerSaturationLimit=0  ZeroCross=off
  Integrator2 : Integrator  UpperSaturationLimit=Inf  LowerSaturationLimit=0  ZeroCross=off
  Phase To Workspace : ToWorkspace  VariableName=result__phase_engine_running_time_secs  SampleTime=-1
  Product1 : Product  Multiplication=Matrix(*)
  Reshape : Reshape
  Total To Workspace : ToWorkspace  VariableName=result__total_engine_running_time_secs  SampleTime=-1
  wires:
  Reshape/1 -> Integrator1/1, Product1/1
  Data Type Conversion/1 -> Reshape/1
  Integrator2/1 -> Phase To Workspace/1
  [REVS_phase_flag] -> Product1/2
  Product1/1 -> Integrator2/1
  Integrator1/1 -> Total To Workspace/1
  in/1 -> Data Type Conversion/1

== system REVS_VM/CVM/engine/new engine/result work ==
  torque_Nm : Inport
  speed_radps : Inport  Port=2
  upstream_iner_kgm2 : Inport  Port=3
  Derivative : Derivative  CoefficientInTFapproximation=1e6
  Gain : Gain  Gain=1/1000
  Integrator1 : Integrator  UpperSaturationLimit=Inf  LowerSaturationLimit=0  ZeroCross=off
  Integrator2 : Integrator  UpperSaturationLimit=Inf  LowerSaturationLimit=0  ZeroCross=off
  Phase To Workspace : ToWorkspace  VariableName=result__phase_crankshaft_output_pos_work_kJ  SampleTime=-1
  Pos : Fcn  Expr=u(1)*(u(1) >= 0)
  Product : Product
  Product1 : Product
  Product2 : Product
  Subtract : Sum  Inputs=+-
  Total To Workspace : ToWorkspace  VariableName=result__total_crankshaft_output_pos_work_kJ  SampleTime=-1
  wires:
  Product2/1 -> Pos/1
  Pos/1 -> Gain/1
  Gain/1 -> Integrator1/1, Product/2
  Product1/1 -> Subtract/2
  Derivative/1 -> Product1/1
  speed_radps/1 -> Derivative/1, Product2/2
  upstream_iner_kgm2/1 -> Product1/2
  Subtract/1 -> Product2/1
  Integrator2/1 -> Phase To Workspace/1
  [REVS_phase_flag] -> Product/1
  Product/1 -> Integrator2/1
  Integrator1/1 -> Total To Workspace/1
  torque_Nm/1 -> Subtract/1

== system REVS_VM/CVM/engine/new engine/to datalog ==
  Var : Inport
  Constant : Constant  Value=VerboseSignal
  Constant1 : Constant  Value=VerboseLevel
  Relational Operator : RelationalOperator  OutDataTypeStr=boolean  ZeroCross=off
  Subsystem : Subsystem
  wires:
  Constant1/1 -> Relational Operator/2
  Constant/1 -> Relational Operator/1
  Relational Operator/1 -> Subsystem/Enable
  Var/1 -> Subsystem/1(In1)

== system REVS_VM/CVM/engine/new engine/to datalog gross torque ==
  Var : Inport
  Constant : Constant  Value=VerboseSignal
  Constant1 : Constant  Value=VerboseLevel
  Relational Operator : RelationalOperator  OutDataTypeStr=boolean  ZeroCross=off
  Subsystem : Subsystem
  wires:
  Constant1/1 -> Relational Operator/2
  Constant/1 -> Relational Operator/1
  Relational Operator/1 -> Subsystem/Enable
  Var/1 -> Subsystem/1(In1)

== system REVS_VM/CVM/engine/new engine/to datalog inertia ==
  Var : Inport
  Constant : Constant  Value=VerboseSignal
  Constant1 : Constant  Value=VerboseLevel
  Relational Operator : RelationalOperator  OutDataTypeStr=boolean  ZeroCross=off
  Subsystem : Subsystem
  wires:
  Constant1/1 -> Relational Operator/2
  Constant/1 -> Relational Operator/1
  Relational Operator/1 -> Subsystem/Enable
  Var/1 -> Subsystem/1(In1)

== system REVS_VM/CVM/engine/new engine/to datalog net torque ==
  Var : Inport
  Constant : Constant  Value=VerboseSignal
  Constant1 : Constant  Value=VerboseLevel
  Relational Operator : RelationalOperator  OutDataTypeStr=boolean  ZeroCross=off
  Subsystem : Subsystem
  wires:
  Constant1/1 -> Relational Operator/2
  Constant/1 -> Relational Operator/1
  Relational Operator/1 -> Subsystem/Enable
  Var/1 -> Subsystem/1(In1)

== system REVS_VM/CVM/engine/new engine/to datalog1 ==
  Var : Inport
  Constant : Constant  Value=VerboseSignal
  Constant1 : Constant  Value=VerboseLevel
  Relational Operator : RelationalOperator  OutDataTypeStr=boolean  ZeroCross=off
  Subsystem : Subsystem
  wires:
  Constant1/1 -> Relational Operator/2
  Constant/1 -> Relational Operator/1
  Relational Operator/1 -> Subsystem/Enable
  Var/1 -> Subsystem/1(In1)

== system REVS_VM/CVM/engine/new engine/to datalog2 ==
  Var : Inport
  Constant : Constant  Value=VerboseSignal
  Constant1 : Constant  Value=VerboseLevel
  Relational Operator : RelationalOperator  OutDataTypeStr=boolean  ZeroCross=off
  Subsystem : Subsystem
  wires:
  Constant1/1 -> Relational Operator/2
  Constant/1 -> Relational Operator/1
  Relational Operator/1 -> Subsystem/Enable
  Var/1 -> Subsystem/1(In1)

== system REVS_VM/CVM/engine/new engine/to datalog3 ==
  Var : Inport
  Constant : Constant  Value=VerboseSignal
  Constant1 : Constant  Value=VerboseLevel
  Relational Operator : RelationalOperator  OutDataTypeStr=boolean  ZeroCross=off
  Subsystem : Subsystem
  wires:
  Constant1/1 -> Relational Operator/2
  Constant/1 -> Relational Operator/1
  Relational Operator/1 -> Subsystem/Enable
  Var/1 -> Subsystem/1(In1)

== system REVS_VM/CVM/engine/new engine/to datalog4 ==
  Var : Inport
  Constant : Constant  Value=VerboseSignal
  Constant1 : Constant  Value=VerboseLevel
  Relational Operator : RelationalOperator  OutDataTypeStr=boolean  ZeroCross=off
  Subsystem : Subsystem
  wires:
  Constant1/1 -> Relational Operator/2
  Constant/1 -> Relational Operator/1
  Relational Operator/1 -> Subsystem/Enable
  Var/1 -> Subsystem/1(In1)

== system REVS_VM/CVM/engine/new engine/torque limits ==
  eng_on : Inport
  eng_spd_radps : Inport  Port=2
  Closed Throttle Torque : Lookup_n-D  NumberOfTableDimensions=1  BreakpointsForDimension1=engine.closed_throttle_speed_radps  BeginIndexSearchUsingPreviousIndexResult=on  Table=engine.closed_throttle_torque_Nm  ExtrapMethod=Clip  UseLastTableValue=on  RndMeth=Simplest
  Full Throttle Torque : Lookup_n-D  NumberOfTableDimensions=1  BreakpointsForDimension1=engine.full_throttle_speed_radps  BeginIndexSearchUsingPreviousIndexResult=on  Table=engine.full_throttle_torque_Nm  ExtrapMethod=Clip  UseLastTableValue=on  RndMeth=Simplest
  Product4 : Product  Inputs=3
  to datalog3 : Subsystem
  to datalog4 : Subsystem
  to datalog5 : Subsystem
  current_max_pwr_W : Outport
  current_max_trq_Nm : Outport  Port=2
  current_min_trq_Nm : Outport  Port=3
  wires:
  Closed Throttle Torque/1 -> to datalog5/1(Var), current_min_trq_Nm/1
  eng_on/1 -> Product4/1
  eng_spd_radps/1 -> Full Throttle Torque/1, Closed Throttle Torque/1, Product4/2
  Product4/1 -> to datalog3/1(Var), current_max_pwr_W/1
  Full Throttle Torque/1 -> Product4/3, to datalog4/1(Var), current_max_trq_Nm/1

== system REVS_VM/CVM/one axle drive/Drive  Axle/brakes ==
  note: if brakes applied, subtract upstream torques from desired net - reduces brakes for regen, increases if positive torques
  note: speed positive, brakes are negative
  note: speed negative, brakes are positive
  system_bus : Inport
  trq_in_Nm : Inport  Port=2
  spd_in_radps : Inport  Port=3
  Axle Inertia (kg-m^2) : Constant  Value=brake.inertia_kgm2
  Bus Selector : BusSelector  OutputSignals=driver.driver_brk_norm,driver.cycle_spd_mps
  Compare To Zero3 : simulink/Logic and Bit Operations/Compare To Zero  relop===  OutDataTypeStr=boolean
  Compare To Zero4 : simulink/Logic and Bit Operations/Compare To Zero  relop=<=  OutDataTypeStr=boolean
  Compare To Zero : simulink/Logic and Bit Operations/Compare To Zero  relop=>  OutDataTypeStr=boolean
  Compare To Zero1 : simulink/Logic and Bit Operations/Compare To Zero  relop=>  OutDataTypeStr=boolean
  Compare To Zero2 : simulink/Logic and Bit Operations/Compare To Zero  relop=<  OutDataTypeStr=boolean
  Constant1 : Constant
  Data Type Conversion1 : DataTypeConversion
  Data Type Conversion2 : DataTypeConversion
  Gain : Gain  Gain=brake.max_torque_Nm
  Gain1 : Gain  Gain=-brake.max_torque_Nm
  Gain2 : Gain  Gain=-brake.max_torque_Nm
  Gain3 : Gain  Gain=-1
  Logical Operator : Logic  AllPortsSameDT=off  OutDataTypeStr=boolean
  Mech E&P Nm radps : Subsystem
  MinMax : MinMax  Inputs=2  ZeroCross=off
  MinMax1 : MinMax  Function=max  Inputs=2  ZeroCross=off
  MinMax2 : MinMax  Function=max  Inputs=2  ZeroCross=off
  MinMax3 : MinMax  Inputs=2  ZeroCross=off
  Product1 : Product
  Product2 : Product
  Rate Limiter : RateLimiter  RisingSlewLimit=brake.max_torque_Nm  FallingSlewLimit=-brake.max_torque_Nm
  Sign : Lookup_n-D  NumberOfTableDimensions=1  BreakpointsForDimension1=[-eps 0 eps]  BeginIndexSearchUsingPreviousIndexResult=on  Table=[-1 1 1]  ExtrapMethod=Clip  UseLastTableValue=on  RndMeth=Simplest
  Sum : Sum  Inputs=+-
  Switch : Switch  Criteria=u2 > Threshold
  neg lim : Gain  Gain=-brake.max_torque_Nm
  pos lim : Gain  Gain=brake.max_torque_Nm
  trq_out_Nm : Outport
  iner_out_kgm2 : Outport  Port=2
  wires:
  Data Type Conversion2/1 -> Gain1/1
  Data Type Conversion1/1 -> Gain/1
  Gain1/1 -> MinMax1/2
  Compare To Zero2/1 -> Data Type Conversion2/1
  Gain/1 -> MinMax/1
  Compare To Zero1/1 -> Data Type Conversion1/1
  Sum/1 -> MinMax/2
  Product2/1 -> Gain3/1, Sum/2
  Compare To Zero/1 -> Product2/1
  trq_in_Nm/1 -> Product2/2
  Bus Selector/1 -> Gain2/1, Compare To Zero/1  "<driver_brk_norm>"
  spd_in_radps/1 -> Sign/1, Compare To Zero3/1, Mech E&P Nm radps/2(spd_radps)
  Axle Inertia (kg-m^2)/1 -> Mech E&P Nm radps/3(iner_kgm2), iner_out_kgm2/1
  system_bus/1 -> Bus Selector/1
  Sign/1 -> Product1/2
  Gain2/1 -> Product1/1
  MinMax/1 -> MinMax1/1
  Rate Limiter/1 -> trq_out_Nm/1, Mech E&P Nm radps/1(" trq_Nm")
  Compare To Zero3/1 -> Logical Operator/1
  Compare To Zero4/1 -> Logical Operator/2
  Bus Selector/2 -> Compare To Zero4/1  "<cycle_spd_mps>"
  Product1/1 -> Compare To Zero1/1, Sum/1, Compare To Zero2/1  "desired_net_torque vector"
  Logical Operator/1 -> Switch/2
  MinMax1/1 -> Switch/3
  pos lim/1 -> MinMax3/1
  Gain3/1 -> MinMax3/2
  neg lim/1 -> MinMax2/2
  MinMax3/1 -> MinMax2/1
  MinMax2/1 -> Switch/1
  Switch/1 -> Rate Limiter/1
  Constant1/1 -> neg lim/1, pos lim/1

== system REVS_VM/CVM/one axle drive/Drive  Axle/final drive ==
  trq_in_Nm : Inport
  iner_in_kgm2 : Inport  Port=2
  spd_out_radps : Inport  Port=3
  Eff : Subsystem
  Efficiency : Constant  Value=final_drive.efficiency_norm
  Final Drive Gear Ratio : Constant  Value=final_drive.gear_ratio
  Final Drive Inertia : Constant  Value=final_drive.inertia_kgm2
  Input Output Mech E&P Nm radps : Subsystem
  Math Function : Math  Operator=square
  Product : Product
  Product1 : Product
  Product3 : Product
  Sum : Sum
  zero : Constant  Value=0
  trq_out_Nm : Outport
  iner_out_kgm2 : Outport  Port=2
  spd_in_radps : Outport  Port=3
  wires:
  zero/1 -> Input Output Mech E&P Nm radps/3(iner_in_kgm2)
  Eff/1(Output) -> Product/1
  Efficiency/1 -> Eff/1(Efficiency)
  Product3/1 -> spd_in_radps/1, Input Output Mech E&P Nm radps/2(spd_in_radps)
  spd_out_radps/1 -> Product3/2, Input Output Mech E&P Nm radps/5(spd_out_radps)
  Math Function/1 -> Product1/1
  Final Drive Gear Ratio/1 -> Product3/1, Math Function/1, Product/2
  trq_in_Nm/1 -> Input Output Mech E&P Nm radps/1(trq_in_Nm), Eff/2(Input)
  iner_in_kgm2/1 -> Product1/2
  Product1/1 -> Sum/1
  Final Drive Inertia/1 -> Sum/2, Input Output Mech E&P Nm radps/6(iner_out_kgm2)
  Product/1 -> trq_out_Nm/1, Input Output Mech E&P Nm radps/4(trq_out_Nm)
  Sum/1 -> iner_out_kgm2/1

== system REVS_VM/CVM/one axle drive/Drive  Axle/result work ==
  torque_Nm : Inport
  speed_radps : Inport  Port=2
  upstream_iner_kgm2 : Inport  Port=3
  Derivative : Derivative  CoefficientInTFapproximation=1e6
  Gain : Gain  Gain=1/1000
  Integrator1 : Integrator  UpperSaturationLimit=Inf  LowerSaturationLimit=0  ZeroCross=off
  Integrator2 : Integrator  UpperSaturationLimit=Inf  LowerSaturationLimit=0  ZeroCross=off
  Phase To Workspace : ToWorkspace  VariableName=result__phase_axle_output_pos_work_kJ  SampleTime=-1
  Pos : Fcn  Expr=u(1)*(u(1) >= 0)
  Product : Product
  Product1 : Product
  Product2 : Product
  Subtract : Sum  Inputs=+-
  Total To Workspace : ToWorkspace  VariableName=result__total_axle_output_pos_work_kJ  SampleTime=-1
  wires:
  Product2/1 -> Pos/1
  Pos/1 -> Gain/1
  Gain/1 -> Integrator1/1, Product/2
  Product1/1 -> Subtract/2
  Derivative/1 -> Product1/1
  speed_radps/1 -> Derivative/1, Product2/2
  upstream_iner_kgm2/1 -> Product1/2
  Subtract/1 -> Product2/1
  Integrator2/1 -> Phase To Workspace/1
  [REVS_phase_flag] -> Product/1
  Product/1 -> Integrator2/1
  Integrator1/1 -> Total To Workspace/1
  torque_Nm/1 -> Subtract/1

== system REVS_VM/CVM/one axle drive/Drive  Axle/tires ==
  system_bus : Inport
  trq_in_Nm : Inport  Port=2
  iner_in_kgm2 : Inport  Port=3
  spd_out_mps : Inport  Port=4
  -1..1 : Saturate  UpperLimit=1  LowerLimit=-1  ZeroCross=off
  > 0 : Saturate  UpperLimit=Inf  LowerLimit=0  ZeroCross=off
  Axle Speed (rad/sec) : Product  Inputs=/*
  Compare To Constant : simulink/Logic and Bit Operations/Compare To Constant  relop=>=  const=0.1  OutDataTypeStr=boolean
  Constant : Constant  Value=0
  Dynamic Mass (kg) : Product  Inputs=/*
  Gain : Gain  Gain=-1
  Gain2 : Gain  Gain=100
  Input Output Mech E&P Nm radps N mps : Subsystem
  Math Function : Math  Operator=square
  Mech E&P N mps : Subsystem
  Product : Product  Inputs=3
  Product1 : Product  Inputs=*/
  Sum1 : Sum
  Sum2 : Sum  Inputs=|++
  Tire Inertia (kg-m^2) : Constant  Value=tire.inertia_kgm2
  Tire Radius (m) : Constant  Value=tire.radius_m
  Traction Force (N) : Sum
  Vehicle Weight Fraction : Gain  Gain=tire.vehicle_weight_norm
  const : Constant  Value=vehicle.use_abc_roadload
  normalize : Gain  Gain=1/(eps + tire.wheel_slip_torque_Nm)
  normalized torque to slip norm : Lookup_n-D  NumberOfTableDimensions=1  BreakpointsForDimension1=[-0.999866216844745 -0.99978414282011 -0.99807408909811 -0.994136683198638 -0.987125284420945 -0.975823606608682 -0.958455233159564 -0.932389621966496 -0.893705646328621 -0.836611821621369 -0.752906045607232 -0.632208437687154 -0.464747309940849 -0.248771439727253 0 0.248771439727253 0.464747309940849 0.632208437687154 0.752906045607232 0.836611821621369 0.893705646328621 0.932389621966496 0.95845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  IndexSearchMethod=Linear search  BeginIndexSearchUsingPreviousIndexResult=on  Table=-0.14 : 0.01 : 0.14  ExtrapMethod=Clip  UseLastTableValue=on  RndMeth=Simplest
  numerical stabilizer : TransferFcn  Denominator=[REVS.sim_step_time_secs 1]
  road load sw : Switch  Criteria=u2 > Threshold  ZeroCross=off
  rolling resistance : Subsystem
  rolling resistance coeff : Constant  Value=tire.rolling_resistance_coefficient
  sat eps : Saturate  UpperLimit=Inf  LowerLimit=eps  ZeroCross=off
  to datalog with base name : Subsystem
  zero : Constant  Value=0
  force_out_N : Outport
  mass_out_kg : Outport  Port=2
  spd_in_radps : Outport  Port=3
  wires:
  system_bus/1 -> rolling resistance/1(system_bus)
  zero/1 -> Input Output Mech E&P Nm radps N mps/6(mass_out_kg)
  Math Function/1 -> Dynamic Mass (kg)/1
  sat eps/1 -> Product1/2, Math Function/1, Axle Speed (rad/sec)/1
  Constant/1 -> road load sw/1
  const/1 -> road load sw/2
  Gain/1 -> road load sw/3
  road load sw/1 -> Traction Force (N)/1, Mech E&P N mps/1(force_N)
  Product1/1 -> Traction Force (N)/2, Input Output Mech E&P Nm radps N mps/4(frc_out_N)
  Tire Radius (m)/1 -> sat eps/1
  iner_in_kgm2/1 -> Sum1/1
  Tire Inertia (kg-m^2)/1 -> Input Output Mech E&P Nm radps N mps/3(iner_in_kgm2), Sum1/2
  Sum1/1 -> Dynamic Mass (kg)/2
  Dynamic Mass (kg)/1 -> mass_out_kg/1
  rolling resistance coeff/1 -> Vehicle Weight Fraction/1
  rolling resistance/1(" roll_res_force_N") -> Gain/1
  Vehicle Weight Fraction/1 -> rolling resistance/3(Crr)
  Axle Speed (rad/sec)/1 -> Sum2/1, Product/1
  trq_in_Nm/1 -> Input Output Mech E&P Nm radps N mps/1(trq_in_Nm), normalize/1, Product1/1
  Traction Force (N)/1 -> force_out_N/1
  Product/1 -> numerical stabilizer/1
  Sum2/1 -> Input Output Mech E&P Nm radps N mps/2(spd_in_radps), > 0/1
  numerical stabilizer/1 -> Sum2/2
  spd_out_mps/1 -> Compare To Constant/1, Input Output Mech E&P Nm radps N mps/5(spd_out_mps), Axle Speed (rad/sec)/2, rolling resistance/2(veh_spd_mps), Mech E&P N mps/2(spd_mps)
  > 0/1 -> spd_in_radps/1
  Gain2/1 -> to datalog with base name/1(Var)
  normalize/1 -> -1..1/1
  Compare To Constant/1 -> Product/2
  -1..1/1 -> normalized torque to slip norm/1
  normalized torque to slip norm/1 -> Gain2/1, Product/3

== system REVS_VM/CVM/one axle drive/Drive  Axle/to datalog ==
  Var : Inport
  Constant : Constant  Value=VerboseSignal
  Constant1 : Constant  Value=VerboseLevel
  Relational Operator : RelationalOperator  OutDataTypeStr=boolean  ZeroCross=off
  Subsystem : Subsystem
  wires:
  Constant1/1 -> Relational Operator/2
  Constant/1 -> Relational Operator/1
  Relational Operator/1 -> Subsystem/Enable
  Var/1 -> Subsystem/1(In1)

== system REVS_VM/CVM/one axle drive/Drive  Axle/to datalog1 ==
  Var : Inport
  Constant : Constant  Value=VerboseSignal
  Constant1 : Constant  Value=VerboseLevel
  Relational Operator : RelationalOperator  OutDataTypeStr=boolean  ZeroCross=off
  Subsystem : Subsystem
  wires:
  Constant1/1 -> Relational Operator/2
  Constant/1 -> Relational Operator/1
  Relational Operator/1 -> Subsystem/Enable
  Var/1 -> Subsystem/1(In1)

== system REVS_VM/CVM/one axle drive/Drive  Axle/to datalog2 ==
  Var : Inport
  Constant : Constant  Value=VerboseSignal
  Constant1 : Constant  Value=VerboseLevel
  Relational Operator : RelationalOperator  OutDataTypeStr=boolean  ZeroCross=off
  Subsystem : Subsystem
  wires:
  Constant1/1 -> Relational Operator/2
  Constant/1 -> Relational Operator/1
  Relational Operator/1 -> Subsystem/Enable
  Var/1 -> Subsystem/1(In1)
